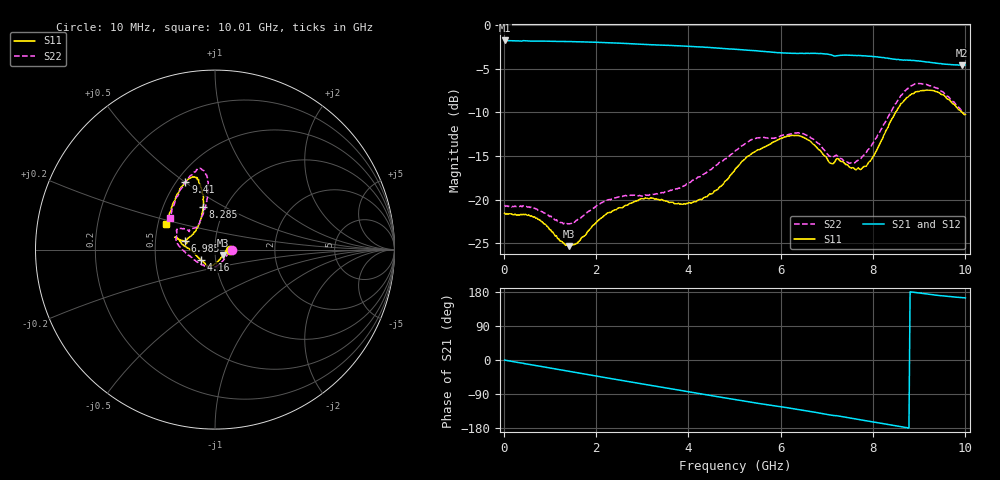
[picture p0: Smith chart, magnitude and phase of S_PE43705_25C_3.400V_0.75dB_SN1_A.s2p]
! Device ID: PE43705
! Serial: 1
! Insertion: A
! Impedance: 50 ohm
! Temp: 25C
! VDD: 3.400V
! Attenuation Step: 0.75dB
#  Hz  S  RI  R  50
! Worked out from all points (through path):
!   401 points, 10 MHz to 10.01 GHz, reference 50 ohm
!   highest |S21| = -1.79 dB at 10 MHz (marker M1); lowest = -4.6 dB at 9.935 GHz (marker M2)
!   group delay of S21, straight-line fit = 55.7 ps
!   lowest |S11| = -25.3 dB at 1.41 GHz (marker M3), VSWR 1.11, Z = 54.6 - j3.32 ohm
!   |S11| at or under -10 dB: start of sweep to 8.497 GHz; 9.936 GHz to end of sweep
!   |S22| runs from -22.8 to -6.7 dB; largest |S21 - S12| = 0.007
!   S11 on the Smith chart (normalised r, x): 10 MHz: 1.18, -0.00; 4.16 GHz: 0.85, -0.09; 6.985 GHz: 0.71, +0.07; 8.285 GHz: 0.79, +0.40; 9.41 GHz: 0.55, +0.50; 10.01 GHz: 0.55, +0.18
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1e7  0.0836 -0.000803  0.8141 -0.00397  0.8145 -0.00384  0.0928 -0.00078
7.1e8  0.0774 0.0119  0.7795 -0.2099  0.7796 -0.2098  0.0882 0.00407
1.41e9  0.0448 -0.0303  0.6956 -0.3999  0.6958 -0.3997  0.0565 -0.0455
1.685e9  0.0279 -0.0539  0.649 -0.4667  0.6489 -0.467  0.0365 -0.0708
2.235e9  -0.00503 -0.0833  0.5354 -0.5812  0.5359 -0.5808  -0.00732 -0.0991
3.36e9  -0.0436 -0.0899  0.2551 -0.7229  0.2558 -0.7225  -0.0628 -0.0882
4.16e9  -0.0798 -0.0555  0.0389 -0.7481  0.0392 -0.7479  -0.12 -0.0523
4.585e9  -0.1086 -0.028  -0.0739 -0.7347  -0.0732 -0.7343  -0.1534 -0.0287
5.01e9  -0.1483 0.00718  -0.1797 -0.7019  -0.1791 -0.7022  -0.1893 0.00702
5.41e9  -0.1836 0.0299  -0.2701 -0.6583  -0.2696 -0.659  -0.2163 0.049
6.085e9  -0.2174 0.0692  -0.3945 -0.5661  -0.3919 -0.5653  -0.2129 0.0977
6.685e9  -0.2021 0.0569  -0.4988 -0.4717  -0.499 -0.4705  -0.1891 0.1189
6.985e9  -0.1685 0.0485  -0.5458 -0.4083  -0.546 -0.4092  -0.1528 0.1092
7.46e9  -0.1391 0.0731  -0.5925 -0.3149  -0.5911 -0.3154  -0.1071 0.1232
7.76e9  -0.1061 0.1065  -0.6189 -0.2452  -0.6177 -0.2473  -0.0853 0.1524
7.985e9  -0.0854 0.1496  -0.6314 -0.192  -0.6306 -0.1954  -0.0674 0.1959
8.285e9  -0.0661 0.238  -0.6339 -0.1212  -0.6335 -0.1248  -0.0446 0.2778
8.36e9  -0.064 0.2644  -0.634 -0.1028  -0.6335 -0.1059  -0.0413 0.3051
8.86e9  -0.0995 0.3913  -0.6256 0.00891  -0.622 0.00463  -0.0724 0.4452
9.41e9  -0.1645 0.3779  -0.594 0.0991  -0.5922 0.0982  -0.1396 0.4105
9.935e9  -0.26 0.1802  -0.5667 0.1554  -0.5694 0.1572  -0.2408 0.2101
1.001e10  -0.2711 0.144  -0.5667 0.1635  -0.5697 0.1631  -0.2531 0.1755
